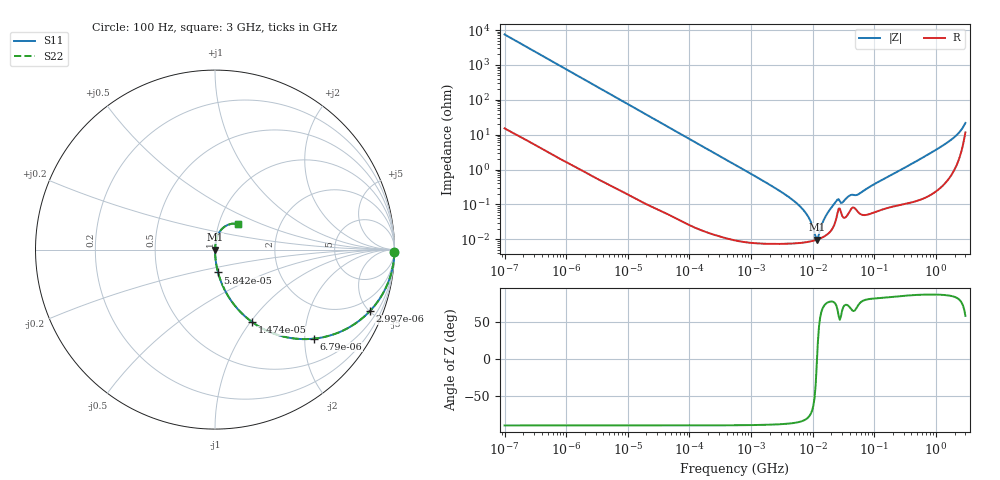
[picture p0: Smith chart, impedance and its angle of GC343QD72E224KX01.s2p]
!Murata Part Number: GC343QD72E224KX01
!These Parameters are Measured in Series Mode Connection
!Data Generated on Jun 10, 2025
!  o--ll--o
!Port1  Port2
!  o------o
!Operation Temp=25[degC], DC Bias Voltage=0[V]
!Freq. Start=100[Hz] Stop=3[GHz] 401[Steps]
# Hz S RI R 50
!Freq.(Hz) S11(Real) S11(Imag) S21(Real) S21(Imag) S12(Real) S12(Imag) S22(Real) S22(Imag)
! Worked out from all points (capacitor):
!   401 points, 100 Hz to 3 GHz, reference 50 ohm
!   read as one part in series: C = 213 nF near 109 Hz
!   lowest |Z| = 9.83 mohm at 11.63 MHz (marker M1)
!   series resonance near 11.75 MHz, so ESL is about 860 pH
!   S11 on the Smith chart (normalised r, x): 100 Hz: open; 2.997 kHz: 1.01, -5.01; 6.79 kHz: 1.01, -2.22; 14.74 kHz: 1.00, -1.02; 58.42 kHz: 1.00, -0.26; 3 GHz: 1.23, +0.37
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100  0.9998 -0.0134  0.000206 0.0134  0.000206 0.0134  0.9998 -0.0134
536  0.9948 -0.0711  0.00524 0.0711  0.00524 0.0711  0.9948 -0.0711
1788  0.9458 -0.2252  0.0542 0.2252  0.0542 0.2252  0.9458 -0.2252
2997  0.8621 -0.3436  0.1379 0.3436  0.1379 0.3436  0.8621 -0.3436
6790  0.5508 -0.4962  0.4492 0.4962  0.4492 0.4962  0.5508 -0.4962
14736  0.2077 -0.4044  0.7923 0.4044  0.7923 0.4044  0.2077 -0.4044
31977  0.0533 -0.2231  0.9467 0.2231  0.9467 0.2231  0.0533 -0.2231
58416  0.0168 -0.127  0.9832 0.127  0.9832 0.127  0.0168 -0.127
547723  0.000284 -0.0138  0.9997 0.0138  0.9997 0.0138  0.000284 -0.0138
4711951  7.78e-05 -0.00135  0.9999 0.00135  0.9999 0.00135  7.78e-05 -0.00135
7565221  8.25e-05 -0.000591  0.9999 0.000591  0.9999 0.000591  8.25e-05 -0.000591
9794414  8.96e-05 -0.000239  0.9999 0.000239  0.9999 0.000239  8.96e-05 -0.000239
1.163455e7  9.75e-05 -1.26e-05  0.9999 1.26e-05  0.9999 1.26e-05  9.75e-05 -1.26e-05
1.268047e7  0.000103 0.000101  0.9999 -0.000101  0.9999 -0.000101  0.000103 0.000101
1.641694e7  0.000131 0.000462  0.9999 -0.000462  0.9999 -0.000462  0.000131 0.000462
2.418395e7  0.000406 0.00121  0.9996 -0.00121  0.9996 -0.00121  0.000406 0.00121
3.131008e7  0.000425 0.00113  0.9996 -0.00113  0.9996 -0.00113  0.000425 0.00113
3.882828e7  0.000593 0.00165  0.9994 -0.00165  0.9994 -0.00165  0.000593 0.00165
5.478864e7  0.000602 0.00186  0.9994 -0.00186  0.9994 -0.00186  0.000602 0.00186
1.751444e8  0.000862 0.00649  0.9991 -0.00649  0.9991 -0.00649  0.000862 0.00649
1.382454e9  0.00667 0.0523  0.9933 -0.0523  0.9933 -0.0523  0.00667 0.0523
3e9  0.1278 0.1438  0.8722 -0.1438  0.8722 -0.1438  0.1278 0.1438
